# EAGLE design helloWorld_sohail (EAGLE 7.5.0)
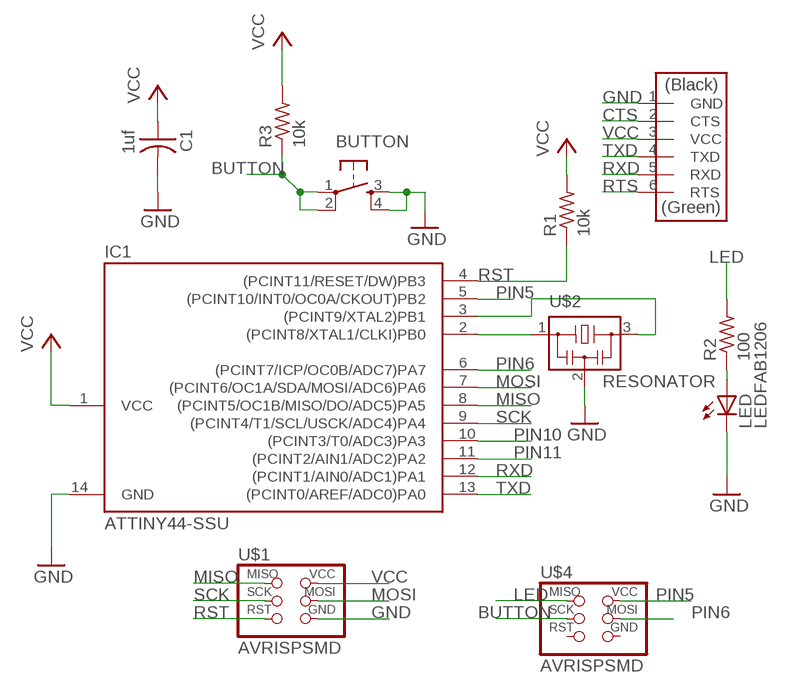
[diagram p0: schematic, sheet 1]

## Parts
BUTTON  6MM_SWITCH6MM_SWITCH  [6MM_SWITCH]
C1  1uf  CAP-US1206FAB  [C1206FAB]
IC1  ATTINY44-SSU  [SOIC14]
LED  LEDFAB1206  [LED1206FAB]
R1  10k  RES-US1206  [R1206]
R2  100  RES-US1206  [R1206]
R3  10k  RES-US1206  [R1206]
U$1  AVRISPSMD  [2X03SMD]
U$2  RESONATOR  [EFOBM]
U$3  FTDI-SMD-HEADER  [1X06SMD]
U$4  AVRISPSMD  [2X03SMD]

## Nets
BUTTON: BUTTON.1(P) BUTTON.2(P1) R3.1 U$4.3(SCK)
CTS: U$3.2(CTS)
GND: BUTTON.3(S) BUTTON.4(S1) C1.2 IC1.14(GND) LED.2(C) U$1.6(GND) U$2.2 U$3.1(GND)
LED: R2.2 U$4.1(MISO)
MISO: IC1.8((PCINT5/OC1B/MISO/DO/ADC5)PA5) U$1.1(MISO)
MOSI: IC1.7((PCINT6/OC1A/SDA/MOSI/ADC6)PA6) U$1.4(MOSI)
N$2: IC1.2((PCINT8/XTAL1/CLKI)PB0) U$2.1
N$3: IC1.3((PCINT9/XTAL2)PB1) U$2.3
N$4: LED.1(A) R2.1
PIN5: IC1.5((PCINT10/INT0/OC0A/CKOUT)PB2) U$4.2(VCC)
PIN6: IC1.6((PCINT7/ICP/OC0B/ADC7)PA7) U$4.4(MOSI)
PIN10: IC1.10((PCINT3/T0/ADC3)PA3)
PIN11: IC1.11((PCINT2/AIN1/ADC2)PA2)
RST: IC1.4((PCINT11/RESET/DW)PB3) R1.1 U$1.5(RST)
RTS: U$3.6(RTS)
RXD: IC1.12((PCINT1/AIN0/ADC1)PA1) U$3.5(RXD)
SCK: IC1.9((PCINT4/T1/SCL/USCK/ADC4)PA4) U$1.3(SCK)
TXD: IC1.13((PCINT0/AREF/ADC0)PA0) U$3.4(TXD)
VCC: C1.1 IC1.1(VCC) R1.2 R3.2 U$1.2(VCC) U$3.3(VCC)
Unconnected: U$4.5(RST) U$4.6(GND)

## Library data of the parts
BUTTON = fab:6MM_SWITCH: OMRON SWITCH
C1 = fab:CAP-US
IC1 = fab:ATTINY44
LED = fab:LED: LED
R1-R3 = fab:RES-US: Resistor (US Symbol)
U$1 U$4 = fab:AVRISP
U$2 = fab:RESONATOR
U$3 = fab:FTDI-SMD-HEADER

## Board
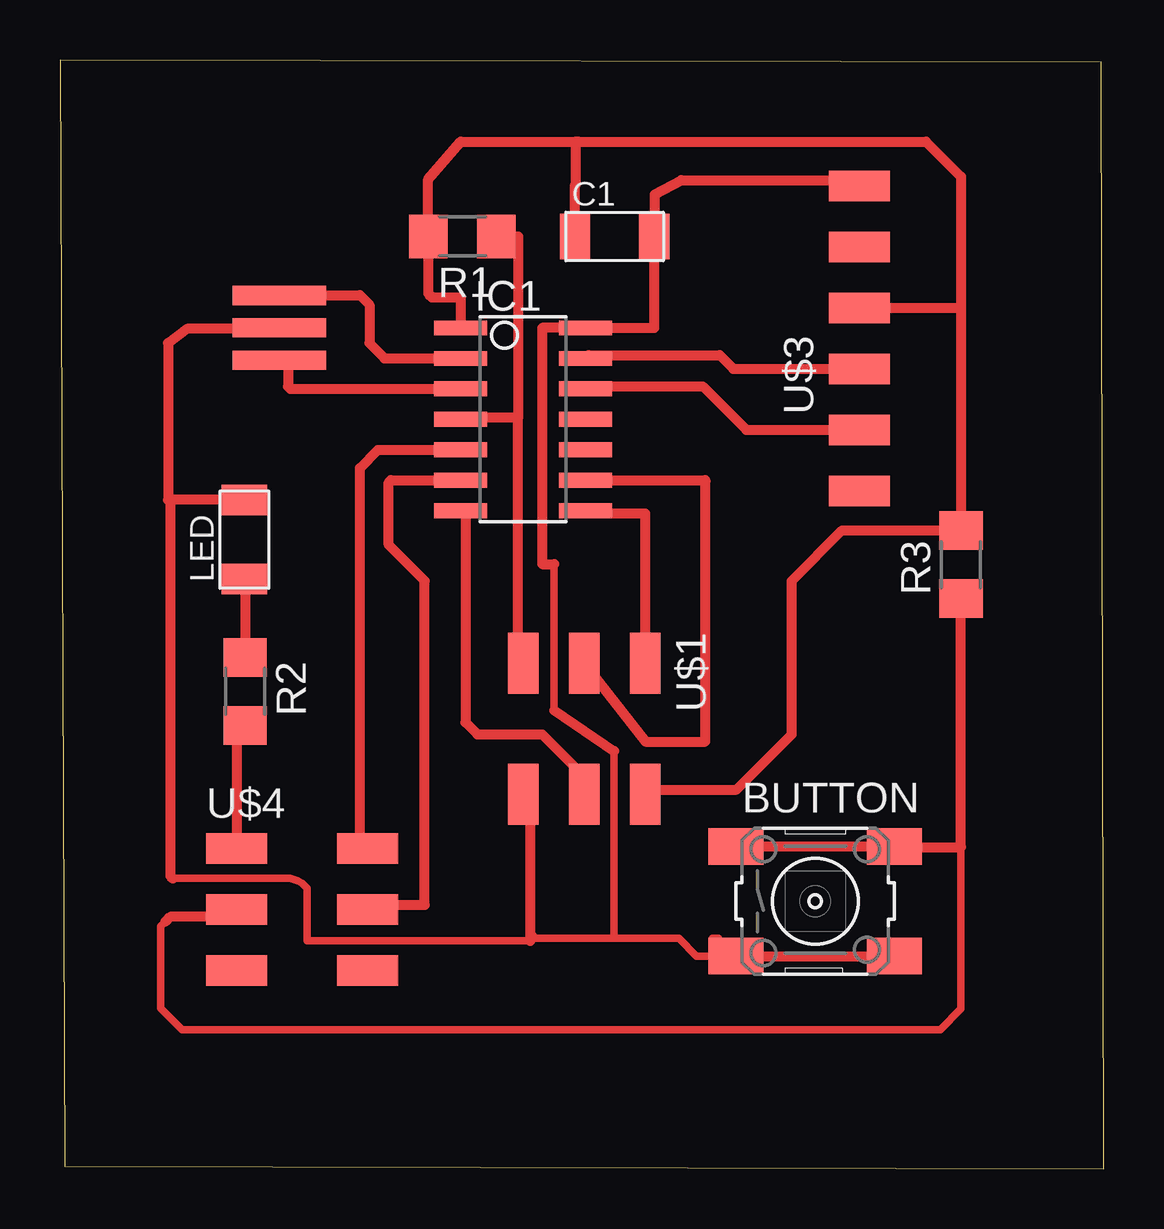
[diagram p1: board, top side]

Size 43.5 x 46.2 mm. Coordinates in mm from the lower left corner, seen from the top.
Outline: 0.2,0.1 43.5,0 43.4,46.1 0,46.2 0.2,0.1
Copper layers (1*16): Top 0.035mm / dielectric 1.5mm / Bottom 0.035mm
Design rules "default *": minimum track width 10mil, minimum drill 24mil, track to track 16mil, track to pad 16mil, pad to pad 16mil, via to via 16mil, smd to smd 16mil, copper to edge 40mil, drill to drill 8mil, minimum pad ring 10mil, minimum via ring 8mil, stop-mask expansion 4mil, vias tented up to drill 0mil, thermal gap 10mil

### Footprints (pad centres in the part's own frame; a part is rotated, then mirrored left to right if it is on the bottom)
6MM_SWITCH = smd 2.286 x 1.524: 1 -3.302,2.286; 2 3.302,2.286; 3 -3.302,-2.286; 4 3.302,-2.286
C1206FAB = smd 1.27 x 1.905: 1 -1.651,0; 2 1.651,0
SOIC14 = smd 0.61 x 2.21: 1 -3.81,-2.603; 2 -2.54,-2.603; 3 -1.27,-2.603; 4 0,-2.603; 5 1.27,-2.603; 6 2.54,-2.603; 7 3.81,-2.603; 8 3.81,2.603; 9 2.54,2.603; 10 1.27,2.603; 11 0,2.603; 12 -1.27,2.603; 13 -2.54,2.603; 14 -3.81,2.603
LED1206FAB = smd 1.27 x 1.905: 1 -1.651,0; 2 1.651,0
R1206 = smd 1.6 x 1.803: 1 -1.422,0; 2 1.422,0
2X03SMD = smd 2.54 x 1.27: 1 -2.54,2.54; 2 2.92,2.54; 3 -2.54,0; 4 2.92,0; 5 -2.54,-2.54; 6 2.92,-2.54
EFOBM = smd 0.8 x 3.9: 1 -1.35,0; 2 0,0; 3 1.35,0
1X06SMD = smd 2.54 x 1.27: 1 0,6.35; 2 0,3.81; 3 0,1.27; 4 0,-1.27; 5 0,-3.81; 6 0,-6.35

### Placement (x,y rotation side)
BUTTON  31.48,11.15 0 top
C1  23.12,38.85 0 top
IC1  19.31,31.23 270 top
LED  7.69,26.22 90 top
R1  16.77,38.85 180 top
R2  7.72,19.89 270 top
R3  37.56,25.18 90 top
U$1  21.85,18.53 270 top
U$2  9.15,35.04 270 top
U$3  33.32,34.6 0 top
U$4  9.9,10.8 0 top

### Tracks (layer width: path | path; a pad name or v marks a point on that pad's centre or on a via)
BUTTON
  Top 0.305: 4.4,10.3 4.2,10.1 4.2,6.7 5.1,5.8 36.7,5.8 37.56,6.66 37.56,13.4
  Top 0.406: BUTTON.1 BUTTON.2 34.82,13.4 37.56,13.4 R3.1 | U$4.3 7.06,10.5 4.6,10.5 4.4,10.3
GND
  Top 0.305: 20.6,25.2 20.6,19.1 | U$2.2 9.11,35 | 23.1,17.4 23.1,9.6 | 23.1,9.6 25.8,9.6 26.54,8.86 27.6,8.86 | 23.1,9.6 19.8,9.6 19.6,9.9 | 4.7,12.1 9.6,12.1 9.9,12 10.1,11.9 10.3,11.7 10.3,9.5 19.6,9.5 | 27.6,8.86 BUTTON.3 | 27.44,9.6 27.2,9.6 27.6,9.2 27.6,8.86
  Top 0.406: U$3.1 32.6,41.2 25.9,41.2 24.8,40.6 C1.2 24.77,35.04 IC1.14 20.1,35.04 20.1,25.2 20.6,25.2 | BUTTON.3 BUTTON.4 | LED.2 4.5,27.87 | 20.6,19.1 23.1,17.4 | 9.11,35 5.3,35 4.5,34.4 4.5,27.87 | 4.5,27.87 4.6,27.77 4.6,12.2 4.7,12.1 | U$1.6 19.6,15.32 19.6,9.9 19.6,9.5
LED
  Top 0.406: R2.2 7.36,18.11 U$4.1
MISO
  Top 0.406: U$1.1 24.4,27.3 21.91,27.3 IC1.8
MOSI
  Top 0.406: 21.6,15.86 U$1.4 22.05,16.15 20.1,18.1 17.4,18.1 16.9,18.6 16.9,27.23 IC1.7
N$2
  Top 0.305: U$2.1
  Top 0.406: U$2.1 12.5,36.4 12.9,36 12.9,34.4 13.53,33.77 IC1.2
N$3
  Top 0.305: U$2.3 9.5,33.34 | 9.5,32.6 9.6,32.5
  Top 0.406: 9.5,33.34 9.5,32.6 | 9.6,32.5 IC1.3
N$4
  Top 0.406: LED.1 7.72,24.54 R2.1
PIN5
  Top 0.406: U$4.2 12.5,13.66 12.5,29.2 13.26,29.96 IC1.5
PIN6
  Top 0.406: U$4.4 13.02,11 15.2,11 15.2,24.5 13.7,26 13.7,28.6 13.79,28.69 IC1.6
RST
  Top 0.406: U$1.5 19.1,21.07 19.1,31.3 | 19.1,31.3 16.71,31.3 IC1.4 | R1.1 19.1,38.85 19.1,31.3
RXD
  Top 0.305: IC1.12 22.01,32.6
  Top 0.406: U$3.5 28.61,30.79 26.8,32.6 22.01,32.6
SCK
  Top 0.406: U$1.3 24.4,17.8 26.9,17.8 26.9,28.4 26.9,28.6 26.9,28.69 IC1.9
TXD
  Top 0.406: IC1.13 22.04,33.9 27.5,33.9 28.07,33.33 U$3.4
VCC
  Top 0.406: C1.1 21.47,41.01 21.5,41.01 21.5,42.8 | IC1.1 16.71,36.31 15.5,36.31 15.35,36.46 R1.2 15.35,41.24 16.7,42.8 21.5,42.8 | 21.5,42.8 21.6,42.79 21.61,42.8 36.1,42.8 37.56,41.34 37.56,35.87 | U$3.3 37.56,35.87 | 37.56,35.87 R3.2 32.6,26.6 30.5,24.5 30.5,18.1 28.2,15.8 24.58,15.8 U$1.2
